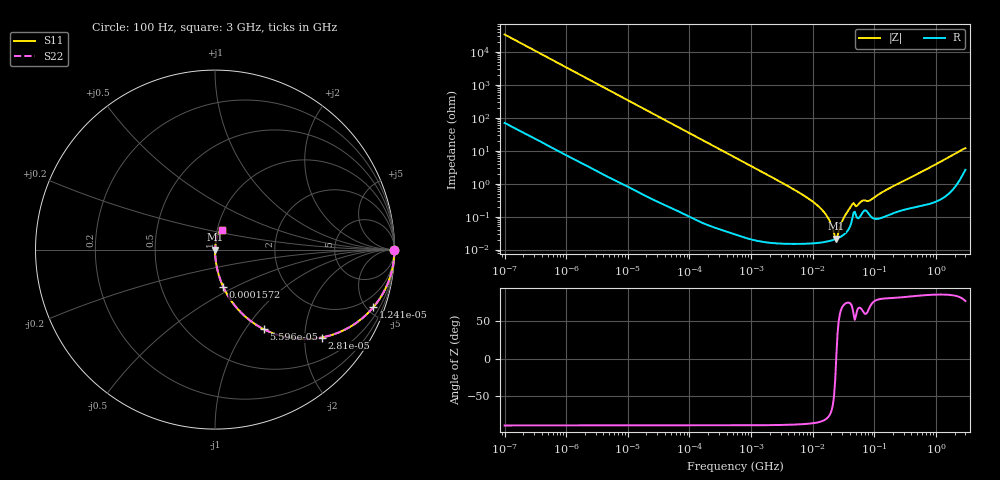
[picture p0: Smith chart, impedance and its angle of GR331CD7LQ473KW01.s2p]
!Murata Part Number: GR331CD7LQ473KW01
!These Parameters are Measured in Series Mode Connection
!Data Generated on Mar 13, 2026
!  o--ll--o
!Port1  Port2
!  o------o
!Operation Temp=25[degC], DC Bias Voltage=0[V]
!Freq. Start=100[Hz] Stop=3[GHz] 401[Steps]
# Hz S RI R 50
!Freq.(Hz) S11(Real) S11(Imag) S21(Real) S21(Imag) S12(Real) S12(Imag) S22(Real) S22(Imag)
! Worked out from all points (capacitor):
!   401 points, 100 Hz to 3 GHz, reference 50 ohm
!   read as one part in series: C = 47.2 nF near 109 Hz
!   lowest |Z| = 21.2 mohm at 24.18 MHz (marker M1)
!   series resonance near 24.06 MHz, so ESL is about 930 pH
!   S11 on the Smith chart (normalised r, x): 100 Hz: open; 12.4 kHz: 1.01, -5.47; 28.1 kHz: 1.01, -2.42; 55.95 kHz: 1.00, -1.22; 157.2 kHz: 1.00, -0.43; 3 GHz: 1.05, +0.23
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100  1 -0.00297  1.49e-05 0.00297  1.49e-05 0.00297  1 -0.00297
1788  0.9971 -0.0527  0.0029 0.0527  0.0029 0.0527  0.9971 -0.0527
5024  0.9782 -0.1449  0.0218 0.1449  0.0218 0.1449  0.9782 -0.1449
12405  0.8816 -0.3219  0.1184 0.3219  0.1184 0.3219  0.8816 -0.3219
28103  0.5937 -0.4899  0.4063 0.4899  0.4063 0.4899  0.5937 -0.4899
31977  0.5305 -0.4978  0.4695 0.4978  0.4695 0.4978  0.5305 -0.4978
55955  0.2705 -0.4429  0.7295 0.4429  0.7295 0.4429  0.2705 -0.4429
157206  0.0455 -0.2068  0.9545 0.2068  0.9545 0.2068  0.0455 -0.2068
547723  0.00415 -0.0621  0.9958 0.0621  0.9958 0.0621  0.00415 -0.0621
9794414  0.000162 -0.00293  0.9998 0.00293  0.9998 0.00293  0.000162 -0.00293
1.641694e7  0.000173 -0.00113  0.9998 0.00113  0.9998 0.00113  0.000173 -0.00113
1.950129e7  0.000185 -0.000612  0.9998 0.000612  0.9998 0.000612  0.000185 -0.000612
2.21892e7  0.000199 -0.000236  0.9998 0.000236  0.9998 0.000236  0.000199 -0.000236
2.418395e7  0.000211 1.53e-05  0.9998 -1.53e-05  0.9998 -1.53e-05  0.000211 1.53e-05
2.52476e7  0.000218 0.000142  0.9998 -0.000142  0.9998 -0.000142  0.000218 0.000142
3.268714e7  0.000293 0.000949  0.9997 -0.000949  0.9997 -0.000949  0.000293 0.000949
4.231884e7  0.000656 0.00202  0.9993 -0.00202  0.9993 -0.00202  0.000656 0.00202
5.248048e7  0.00092 0.00191  0.9991 -0.00191  0.9991 -0.00191  0.00092 0.00191
6.508213e7  0.00137 0.00275  0.9986 -0.00275  0.9986 -0.00275  0.00137 0.00275
8.425944e7  0.0011 0.00286  0.9989 -0.00286  0.9989 -0.00286  0.0011 0.00286
1.751444e8  0.00118 0.00716  0.9988 -0.00716  0.9988 -0.00716  0.00118 0.00716
3e9  0.0379 0.1089  0.9621 -0.1089  0.9621 -0.1089  0.0379 0.1089
